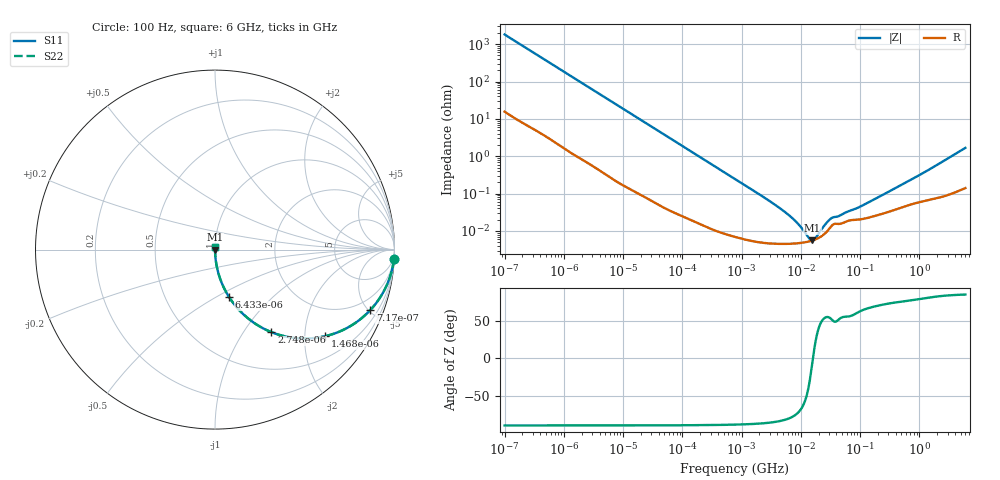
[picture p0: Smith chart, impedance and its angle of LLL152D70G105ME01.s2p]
!Murata Part Number: LLL152D70G105ME01
!These Parameters are Measured in Series Mode Connection
!Data Generated on Jan 08, 2026
!  o--ll--o
!Port1  Port2
!  o------o
!Operation Temp=25[degC], DC Bias Voltage=0[V]
!Freq. Start=100[Hz] Stop=6[GHz] 401[Steps]
# Hz S RI R 50
!Freq.(Hz) S11(Real) S11(Imag) S21(Real) S21(Imag) S12(Real) S12(Imag) S22(Real) S22(Imag)
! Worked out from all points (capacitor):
!   401 points, 100 Hz to 6 GHz, reference 50 ohm
!   read as one part in series: C = 872 nF near 109 Hz
!   lowest |Z| = 5.6 mohm at 15.56 MHz (marker M1)
!   series resonance near 16.02 MHz, so ESL is about 110 pH
!   S11 on the Smith chart (normalised r, x): 100 Hz: 1, -36; 717 Hz: 1.05, -5.13; 1.468 kHz: 1.02, -2.52; 2.748 kHz: 1.01, -1.35; 6.433 kHz: 1.01, -0.58; 6 GHz: 1.00, +0.03
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100  0.9965 -0.0547  0.00348 0.0547  0.00348 0.0547  0.9965 -0.0547
293  0.9737 -0.1555  0.0263 0.1555  0.0263 0.1555  0.9737 -0.1555
717  0.866 -0.3361  0.134 0.3361  0.134 0.3361  0.866 -0.3361
1026  0.7618 -0.4216  0.2382 0.4216  0.2382 0.4216  0.7618 -0.4216
1468  0.6122 -0.4829  0.3878 0.4829  0.3878 0.4829  0.6122 -0.4829
2008  0.4598 -0.4939  0.5402 0.4939  0.5402 0.4939  0.4598 -0.4939
2748  0.3146 -0.4599  0.6854 0.4599  0.6854 0.4599  0.3146 -0.4599
4111  0.172 -0.3729  0.828 0.3729  0.828 0.3729  0.172 -0.3729
6433  0.0794 -0.266  0.9206 0.266  0.9206 0.266  0.0794 -0.266
15062  0.0163 -0.1221  0.9837 0.1221  0.9837 0.1221  0.0163 -0.1221
40335  0.00266 -0.0465  0.9973 0.0465  0.9973 0.0465  0.00266 -0.0465
774597  7.55e-05 -0.00248  0.9999 0.00248  0.9999 0.00248  7.55e-05 -0.00248
4856642  4.52e-05 -0.000363  1 0.000363  1 0.000363  4.52e-05 -0.000363
7266822  4.58e-05 -0.000213  1 0.000213  1 0.000213  4.58e-05 -0.000213
1.137099e7  4.94e-05 -8.51e-05  1 8.51e-05  1 8.51e-05  4.94e-05 -8.51e-05
1.555665e7  5.55e-05 -7.2e-06  0.9999 7.2e-06  0.9999 7.2e-06  5.55e-05 -7.2e-06
2.035112e7  6.63e-05 5.94e-05  0.9999 -5.94e-05  0.9999 -5.94e-05  6.63e-05 5.94e-05
3.330331e7  0.000138 0.000176  0.9999 -0.000176  0.9999 -0.000176  0.000138 0.000176
9.326766e7  0.000201 0.000373  0.9998 -0.000373  0.9998 -0.000373  0.000201 0.000373
3.124326e8  0.000331 0.0011  0.9997 -0.0011  0.9997 -0.0011  0.000331 0.0011
1.197065e9  0.000643 0.00361  0.9994 -0.00361  0.9994 -0.00361  0.000643 0.00361
6e9  0.00169 0.0167  0.9983 -0.0167  0.9983 -0.0167  0.00169 0.0167
